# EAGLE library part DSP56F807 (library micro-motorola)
16-bit Digital Signal Processor
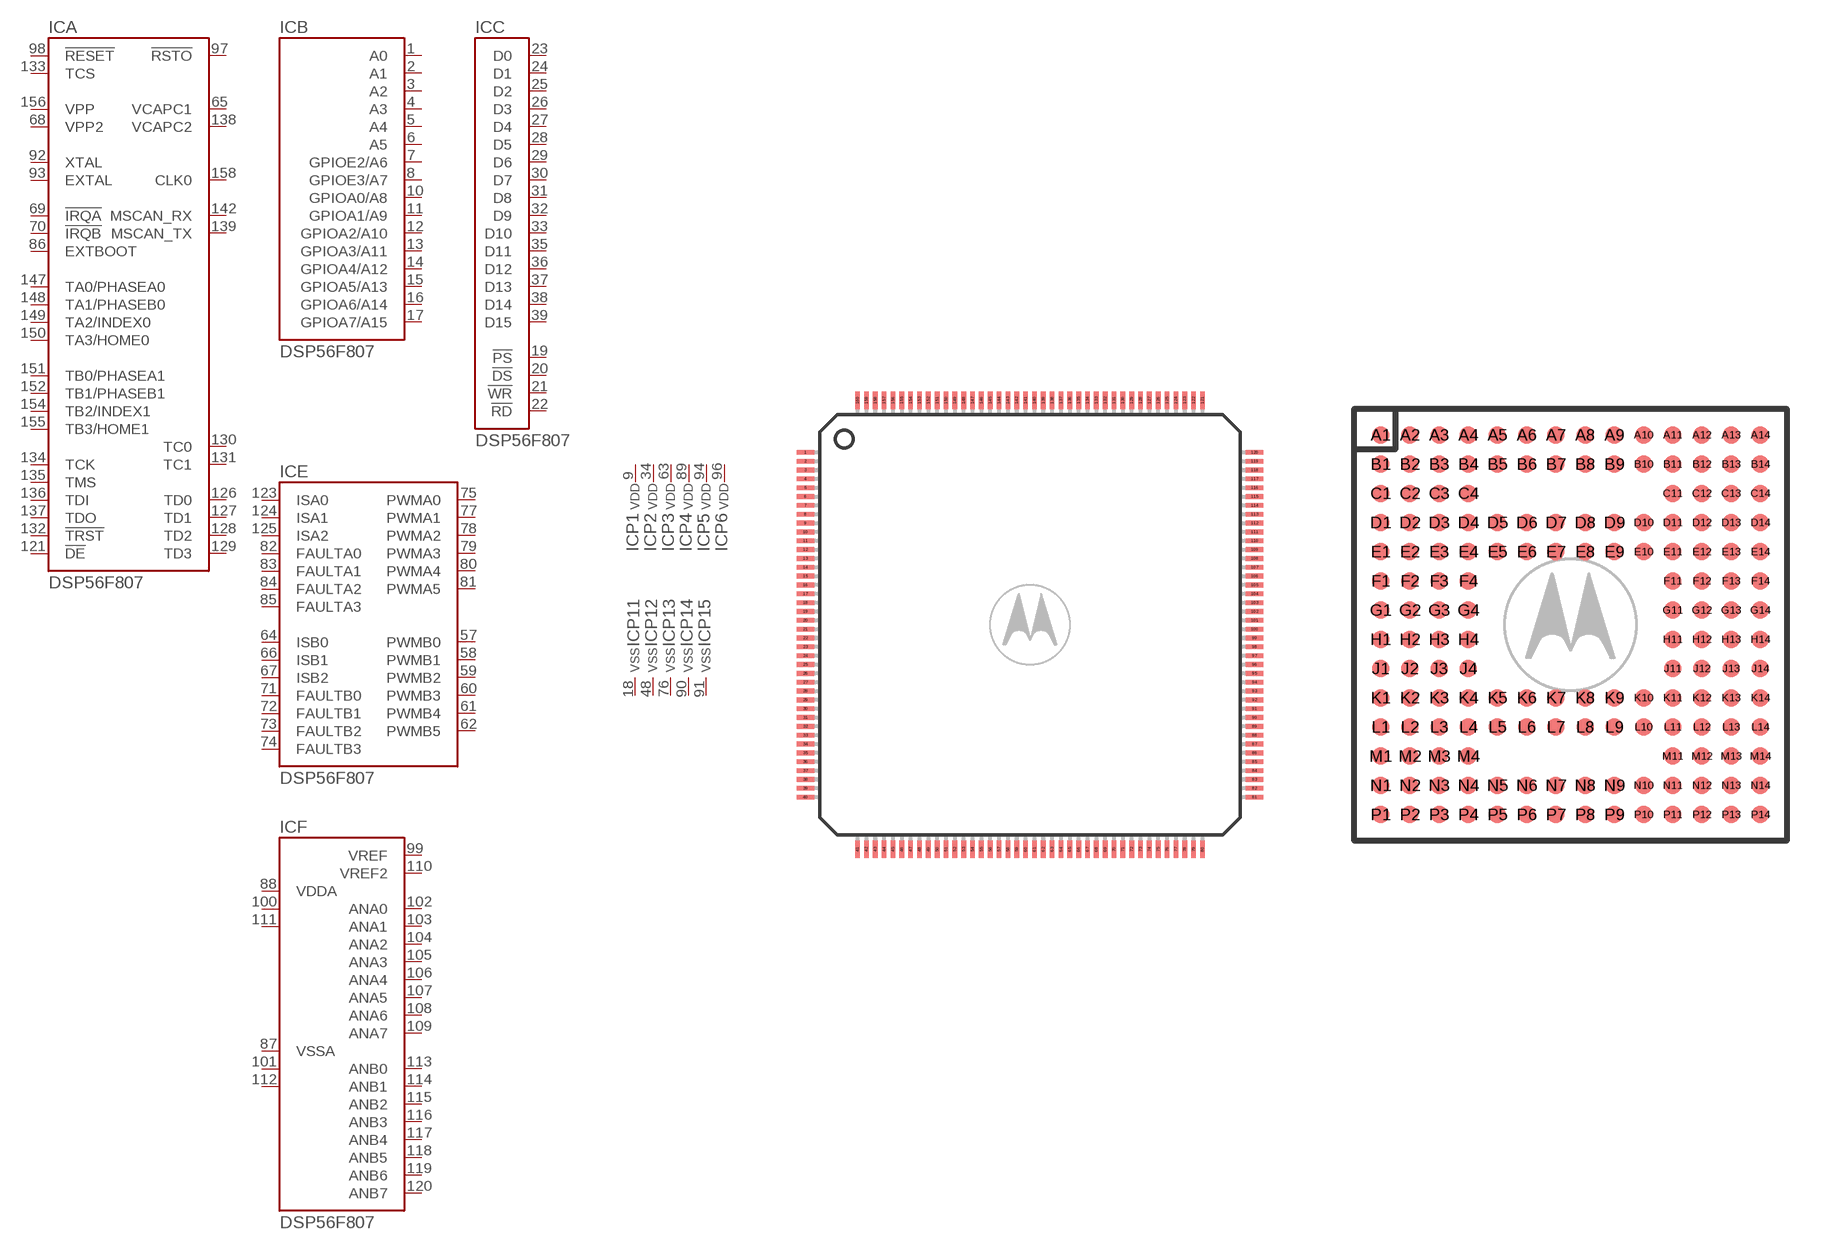
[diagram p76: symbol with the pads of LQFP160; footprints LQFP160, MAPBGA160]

Designator prefix IC; gates A=DSP56F807-CTRL B=DSP56F807-ADR C=DSP56F807-DATA E=DSP56F807-PWM F=DSP56F807-ANA P1=VDD P2=VDD P3=VDD P4=VDD P5=VDD P6=VDD P11=VSS P12=VSS P13=VSS P14=VSS P15=VSS P16=VSS P17=VSS P7=VDD P18=VSS D=DSP56F807-PORT P8=VDD P19=VSS

## DSP56F807PY80 (MF: MOTOROLA; MPN: DSP56F807PY80; OC_FARNELL: 1691514; OC_NEWARK: 74C6821)  [LQFP160]
1  B:A0  out
2  B:A1  out
3  B:A2  out
4  B:A3  out
5  B:A4  out
6  B:A5  out
7  B:GPIOE2/A6
8  B:GPIOE3/A7
9  P1:VDD  pwr
10  B:GPIOA0/A8
11  B:GPIOA1/A9
12  B:GPIOA2/A10
13  B:GPIOA3/A11
14  B:GPIOA4/A12
15  B:GPIOA5/A13
16  B:GPIOA6/A14
17  B:GPIOA7/A15
18  P11:VSS  pwr
19  C:!PS  out
20  C:!DS  out
21  C:!WR  out
22  C:!RD  out
23  C:D0
24  C:D1
25  C:D2
26  C:D3
27  C:D4
28  C:D5
29  C:D6
30  C:D7
31  C:D8
32  C:D9
33  C:D10
34  P2:VDD  pwr
35  C:D11
36  C:D12
37  C:D13
38  C:D14
39  C:D15
40  D:GPIOB0
41  D:GPIOB1
42  D:GPIOB2
43  D:GPIOB3
44  D:GPIOB4
45  D:GPIOB5
46  D:GPIOB6
47  D:GPIOB7
48  P12:VSS  pwr
49  D:GPIOD0
50  D:GPIOD1
51  D:GPIOD2
52  D:GPIOD3
53  D:GPIOD4
54  D:GPIOD5
55  D:GPIOD6/TXD1
56  D:GPIOD7/RXD1
57  E:PWMB0  out
58  E:PWMB1  out
59  E:PWMB2  out
60  E:PWMB3  out
61  E:PWMB4  out
62  E:PWMB5  out
63  P3:VDD  pwr
64  E:ISB0  in
65  A:VCAPC1  out
66  E:ISB1  in
67  E:ISB2  in
68  A:VPP2
69  A:!IRQA  in
70  A:!IRQB  in
71  E:FAULTB0  in
72  E:FAULTB1  in
73  E:FAULTB2  in
74  E:FAULTB3  in
75  E:PWMA0  out
76  P13:VSS  pwr
77  E:PWMA1  out
78  E:PWMA2  out
79  E:PWMA3  out
80  E:PWMA4  out
81  E:PWMA5  out
82  E:FAULTA0  in
83  E:FAULTA1  in
84  E:FAULTA2  in
85  E:FAULTA3  in
86  A:EXTBOOT  in
87  F:VSSA  pwr
88  F:VDDA  pwr
89  P4:VDD  pwr
90  P14:VSS  pwr
91  P15:VSS  pwr
92  A:XTAL
93  A:EXTAL  in
94  P5:VDD  pwr
95  P16:VSS  pwr
96  P6:VDD  pwr
97  A:!RSTO  out
98  A:!RESET  in
99  F:VREF  in
100  F:VDDA  pwr
101  F:VSSA  pwr
102  F:ANA0  in
103  F:ANA1  in
104  F:ANA2  in
105  F:ANA3  in
106  F:ANA4  in
107  F:ANA5  in
108  F:ANA6  in
109  F:ANA7  in
110  F:VREF2  in
111  F:VDDA  pwr
112  F:VSSA  pwr
113  F:ANB0  in
114  F:ANB1  in
115  F:ANB2  in
116  F:ANB3  in
117  F:ANB4  in
118  F:ANB5  in
119  F:ANB6  in
120  F:ANB7  in
121  A:!DE  out
122  P17:VSS  pwr
123  E:ISA0  in
124  E:ISA1  in
125  E:ISA2  in
126  A:TD0
127  A:TD1
128  A:TD2
129  A:TD3
130  A:TC0
131  A:TC1
132  A:!TRST  in
133  A:TCS  pas
134  A:TCK  in
135  A:TMS  in
136  A:TDI  in
137  A:TDO  out
138  A:VCAPC2  out
139  A:MSCAN_TX  out
140  P7:VDD  pwr
141  P18:VSS  pwr
142  A:MSCAN_RX  in
143  D:GPIOE7/!SS
144  D:GPIOE4/SCLK
145  D:GPIOE6/MISO
146  D:GPIOE5/MOSI
147  A:TA0/PHASEA0
148  A:TA1/PHASEB0
149  A:TA2/INDEX0
150  A:TA3/HOME0
151  A:TB0/PHASEA1
152  A:TB1/PHASEB1
153  P8:VDD  pwr
154  A:TB2/INDEX1
155  A:TB3/HOME1
156  A:VPP
157  P19:VSS  pwr
158  A:CLK0  out
159  D:GPIOE0/TXD0
160  D:GPIOE1/RXD0

## DSP56F807VF80 (OC_FARNELL: 1691535; OC_NEWARK: unknown)  [MAPBGA160]
A1  D:GPIOE1/RXD0
A2  A:CLK0  out
A3  P19:VSS  pwr
A4  P8:VDD  pwr
A5  A:TA3/HOME0
A6  D:GPIOE5/MOSI
A7  D:GPIOE7/!SS
A8  A:VCAPC2  out
A9  A:TMS  in
A10  A:TC0
A11  A:TD1
A12  E:ISA2  in
A13  E:ISA1  in
A14  P16:VSS  pwr
B1  B:A4  out
B2  B:A1  out
B3  D:GPIOE0/TXD0
B4  A:VPP
B5  A:TB1/PHASEB1
B6  A:TA2/INDEX0
B7  D:GPIOE6/MISO
B8  A:TDO  out
B9  A:TCS  pas
B10  A:TD3
B11  A:TD0
B12  E:ISA0  in
B13  A:!DE  out
B14  F:ANB6  in
C1  B:GPIOE2/A6
C2  B:A3  out
C3  B:A0  out
C4  A:TB3/HOME1
C11  F:ANB5  in
C12  F:ANB7  in
C13  F:ANB4  in
C14  F:ANB3  in
D1  B:GPIOE3/A7
D2  B:A5  out
D3  B:A2  out
D4  A:TB2/INDEX1
D5  A:TA1/PHASEB0
D6  A:MSCAN_RX  in
D7  P6:VDD  pwr
D8  A:TDI  in
D9  A:!TRST  in
D10  A:TD2
D11  F:ANB0  in
D12  F:ANB1  in
D13  F:ANB2  in
D14  F:VSSA  pwr
E1  B:GPIOA1/A9
E2  B:GPIOA0/A8
E3  P1:VDD  pwr
E4  A:TB0/PHASEA1
E5  D:GPIOE4/SCLK
E6  A:TA0/PHASEA0
E7  P17:VSS  pwr
E8  A:MSCAN_TX  out
E9  A:TCK  in
E10  A:TC1
E11  F:ANA5  in
E12  F:ANA7  in
E13  F:VDDA  pwr
E14  F:VREF2  in
F1  B:GPIOA4/A12
F2  B:GPIOA3/A11
F3  B:GPIOA2/A10
F4  P11:VSS  pwr
F11  F:ANA1  in
F12  F:ANA3  in
F13  F:ANA6  in
F14  F:ANA4  in
G1  B:GPIOA7/A15
G2  B:GPIOA6/A14
G3  B:GPIOA5/A13
G4  C:!PS  out
G11  F:VSSA  pwr
G12  F:VDDA  pwr
G13  F:ANA2  in
G14  F:ANA0  in
H1  C:D1
H2  C:D2
H3  C:D0
H4  C:!DS  out
H11  F:VREF  in
H12  A:!RSTO  out
H13  P5:VDD  pwr
H14  A:!RESET  in
J1  C:D4
J2  C:D5
J3  C:D3
J4  C:!WR  out
J11  P15:VSS  pwr
J12  A:EXTAL  in
J13  A:XTAL
J14  P4:VDD  pwr
K1  C:D7
K2  C:D9
K3  C:D6
K4  C:!RD  out
K5  D:GPIOD2
K6  D:GPIOD5
K7  E:PWMB2  out
K8  E:PWMB4  out
K9  E:ISB1  in
K10  A:VCAPC1  out
K11  P13:VSS  pwr
K12  F:VSSA  pwr
K13  F:VDDA  pwr
K14  P14:VSS  pwr
L1  C:D8
L2  C:D11
L3  C:D10
L4  D:GPIOB0
L5  P12:VSS  pwr
L6  D:GPIOD4
L7  E:PWMB0  out
L8  E:PWMB3  out
L9  P2:VDD  pwr
L10  A:VPP2
L11  E:FAULTB2  in
L12  E:FAULTA1  in
L13  E:FAULTA3  in
L14  P3:VDD  pwr
M1  P7:VDD  pwr
M2  C:D13
M3  C:D15
M4  D:GPIOB7
M11  E:FAULTB3  in
M12  E:PWMA4  out
M13  E:FAULTA0  in
M14  A:EXTBOOT  in
N1  C:D12
N2  C:D14
N3  D:GPIOB2
N4  D:GPIOB5
N5  D:GPIOD0
N6  D:GPIOD3
N7  D:GPIOD7/RXD1
N8  E:ISB0  in
N9  A:!IRQA  in
N10  E:FAULTB1  in
N11  P18:VSS  pwr
N12  E:PWMA2  out
N13  E:PWMA3  out
N14  E:FAULTA2  in
P1  D:GPIOB1
P2  D:GPIOB3
P3  D:GPIOB4
P4  D:GPIOB6
P5  D:GPIOD1
P6  D:GPIOD6/TXD1
P7  E:PWMB1  out
P8  E:PWMB5  out
P9  E:ISB2  in
P10  A:!IRQB  in
P11  E:FAULTB0  in
P12  E:PWMA0  out
P13  E:PWMA1  out
P14  E:PWMA5  out

## Footprint LQFP160 (pad centres in mm)
Low-Profile Quad Flat Pack LQFP 160 CASE 1259-01
smd 1 x 0.27: 1 -12.7,9.75; 2 -12.7,9.25; 3 -12.7,8.75; 4 -12.7,8.25; 5 -12.7,7.75; 6 -12.7,7.25; 7 -12.7,6.75; 8 -12.7,6.25; 9 -12.7,5.75; 10 -12.7,5.25; 11 -12.7,4.75; 12 -12.7,4.25; 13 -12.7,3.75; 14 -12.7,3.25; 15 -12.7,2.75; 16 -12.7,2.25; 17 -12.7,1.75; 18 -12.7,1.25; 19 -12.7,0.75; 20 -12.7,0.25; 21 -12.7,-0.25; 22 -12.7,-0.75; 23 -12.7,-1.25; 24 -12.7,-1.75; 25 -12.7,-2.25; 26 -12.7,-2.75; 27 -12.7,-3.25; 28 -12.7,-3.75; 29 -12.7,-4.25; 30 -12.7,-4.75; 31 -12.7,-5.25; 32 -12.7,-5.75; 33 -12.7,-6.25; 34 -12.7,-6.75; 35 -12.7,-7.25; 36 -12.7,-7.75; 37 -12.7,-8.25; 38 -12.7,-8.75; 39 -12.7,-9.25; 40 -12.7,-9.75; 81 12.7,-9.75; 82 12.7,-9.25; 83 12.7,-8.75; 84 12.7,-8.25; 85 12.7,-7.75; 86 12.7,-7.25; 87 12.7,-6.75; 88 12.7,-6.25; 89 12.7,-5.75; 90 12.7,-5.25; 91 12.7,-4.75; 92 12.7,-4.25; 93 12.7,-3.75; 94 12.7,-3.25; 95 12.7,-2.75; 96 12.7,-2.25; 97 12.7,-1.75; 98 12.7,-1.25; 99 12.7,-0.75; 100 12.7,-0.25; 101 12.7,0.25; 102 12.7,0.75; 103 12.7,1.25; 104 12.7,1.75; 105 12.7,2.25; 106 12.7,2.75; 107 12.7,3.25; 108 12.7,3.75; 109 12.7,4.25; 110 12.7,4.75; 111 12.7,5.25; 112 12.7,5.75; 113 12.7,6.25; 114 12.7,6.75; 115 12.7,7.25; 116 12.7,7.75; 117 12.7,8.25; 118 12.7,8.75; 119 12.7,9.25; 120 12.7,9.75
smd 0.27 x 1: 41 -9.75,-12.7; 42 -9.25,-12.7; 43 -8.75,-12.7; 44 -8.25,-12.7; 45 -7.75,-12.7; 46 -7.25,-12.7; 47 -6.75,-12.7; 48 -6.25,-12.7; 49 -5.75,-12.7; 50 -5.25,-12.7; 51 -4.75,-12.7; 52 -4.25,-12.7; 53 -3.75,-12.7; 54 -3.25,-12.7; 55 -2.75,-12.7; 56 -2.25,-12.7; 57 -1.75,-12.7; 58 -1.25,-12.7; 59 -0.75,-12.7; 60 -0.25,-12.7; 61 0.25,-12.7; 62 0.75,-12.7; 63 1.25,-12.7; 64 1.75,-12.7; 65 2.25,-12.7; 66 2.75,-12.7; 67 3.25,-12.7; 68 3.75,-12.7; 69 4.25,-12.7; 70 4.75,-12.7; 71 5.25,-12.7; 72 5.75,-12.7; 73 6.25,-12.7; 74 6.75,-12.7; 75 7.25,-12.7; 76 7.75,-12.7; 77 8.25,-12.7; 78 8.75,-12.7; 79 9.25,-12.7; 80 9.75,-12.7; 121 9.75,12.7; 122 9.25,12.7; 123 8.75,12.7; 124 8.25,12.7; 125 7.75,12.7; 126 7.25,12.7; 127 6.75,12.7; 128 6.25,12.7; 129 5.75,12.7; 130 5.25,12.7; 131 4.75,12.7; 132 4.25,12.7; 133 3.75,12.7; 134 3.25,12.7; 135 2.75,12.7; 136 2.25,12.7; 137 1.75,12.7; 138 1.25,12.7; 139 0.75,12.7; 140 0.25,12.7; 141 -0.25,12.7; 142 -0.75,12.7; 143 -1.25,12.7; 144 -1.75,12.7; 145 -2.25,12.7; 146 -2.75,12.7; 147 -3.25,12.7; 148 -3.75,12.7; 149 -4.25,12.7; 150 -4.75,12.7; 151 -5.25,12.7; 152 -5.75,12.7; 153 -6.25,12.7; 154 -6.75,12.7; 155 -7.25,12.7; 156 -7.75,12.7; 157 -8.25,12.7; 158 -8.75,12.7; 159 -9.25,12.7; 160 -9.75,12.7

## Footprint MAPBGA160 (pad centres in mm)
Mold Array Process Ball Grid Array MAPBGA 160 CASE 1268-01
smd 0.6 x 0.6: A1 -6.5,6.5; A2 -5.5,6.5; A3 -4.5,6.5; A4 -3.5,6.5; A5 -2.5,6.5; A6 -1.5,6.5; A7 -0.5,6.5; A8 0.5,6.5; A9 1.5,6.5; A10 2.5,6.5; A11 3.5,6.5; A12 4.5,6.5; A13 5.5,6.5; A14 6.5,6.5; B1 -6.5,5.5; B2 -5.5,5.5; B3 -4.5,5.5; B4 -3.5,5.5; B5 -2.5,5.5; B6 -1.5,5.5; B7 -0.5,5.5; B8 0.5,5.5; B9 1.5,5.5; B10 2.5,5.5; B11 3.5,5.5; B12 4.5,5.5; B13 5.5,5.5; B14 6.5,5.5; C1 -6.5,4.5; C2 -5.5,4.5; C3 -4.5,4.5; C4 -3.5,4.5; C11 3.5,4.5; C12 4.5,4.5; C13 5.5,4.5; C14 6.5,4.5; D1 -6.5,3.5; D2 -5.5,3.5; D3 -4.5,3.5; D4 -3.5,3.5; D5 -2.5,3.5; D6 -1.5,3.5; D7 -0.5,3.5; D8 0.5,3.5; D9 1.5,3.5; D10 2.5,3.5; D11 3.5,3.5; D12 4.5,3.5; D13 5.5,3.5; D14 6.5,3.5; E1 -6.5,2.5; E2 -5.5,2.5; E3 -4.5,2.5; E4 -3.5,2.5; E5 -2.5,2.5; E6 -1.5,2.5; E7 -0.5,2.5; E8 0.5,2.5; E9 1.5,2.5; E10 2.5,2.5; E11 3.5,2.5; E12 4.5,2.5; E13 5.5,2.5; E14 6.5,2.5; F1 -6.5,1.5; F2 -5.5,1.5; F3 -4.5,1.5; F4 -3.5,1.5; F11 3.5,1.5; F12 4.5,1.5; F13 5.5,1.5; F14 6.5,1.5; G1 -6.5,0.5; G2 -5.5,0.5; G3 -4.5,0.5; G4 -3.5,0.5; G11 3.5,0.5; G12 4.5,0.5; G13 5.5,0.5; G14 6.5,0.5; H1 -6.5,-0.5; H2 -5.5,-0.5; H3 -4.5,-0.5; H4 -3.5,-0.5; H11 3.5,-0.5; H12 4.5,-0.5; H13 5.5,-0.5; H14 6.5,-0.5; J1 -6.5,-1.5; J2 -5.5,-1.5; J3 -4.5,-1.5; J4 -3.5,-1.5; J11 3.5,-1.5; J12 4.5,-1.5; J13 5.5,-1.5; J14 6.5,-1.5; K1 -6.5,-2.5; K2 -5.5,-2.5; K3 -4.5,-2.5; K4 -3.5,-2.5; K5 -2.5,-2.5; K6 -1.5,-2.5; K7 -0.5,-2.5; K8 0.5,-2.5; K9 1.5,-2.5; K10 2.5,-2.5; K11 3.5,-2.5; K12 4.5,-2.5; K13 5.5,-2.5; K14 6.5,-2.5; L1 -6.5,-3.5; L2 -5.5,-3.5; L3 -4.5,-3.5; L4 -3.5,-3.5; L5 -2.5,-3.5; L6 -1.5,-3.5; L7 -0.5,-3.5; L8 0.5,-3.5; L9 1.5,-3.5; L10 2.5,-3.5; L11 3.5,-3.5; L12 4.5,-3.5; L13 5.5,-3.5; L14 6.5,-3.5; M1 -6.5,-4.5; M2 -5.5,-4.5; M3 -4.5,-4.5; M4 -3.5,-4.5; M11 3.5,-4.5; M12 4.5,-4.5; M13 5.5,-4.5; M14 6.5,-4.5; N1 -6.5,-5.5; N2 -5.5,-5.5; N3 -4.5,-5.5; N4 -3.5,-5.5; N5 -2.5,-5.5; N6 -1.5,-5.5; N7 -0.5,-5.5; N8 0.5,-5.5; N9 1.5,-5.5; N10 2.5,-5.5; N11 3.5,-5.5; N12 4.5,-5.5; N13 5.5,-5.5; N14 6.5,-5.5; P1 -6.5,-6.5; P2 -5.5,-6.5; P3 -4.5,-6.5; P4 -3.5,-6.5; P5 -2.5,-6.5; P6 -1.5,-6.5; P7 -0.5,-6.5; P8 0.5,-6.5; P9 1.5,-6.5; P10 2.5,-6.5; P11 3.5,-6.5; P12 4.5,-6.5; P13 5.5,-6.5; P14 6.5,-6.5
